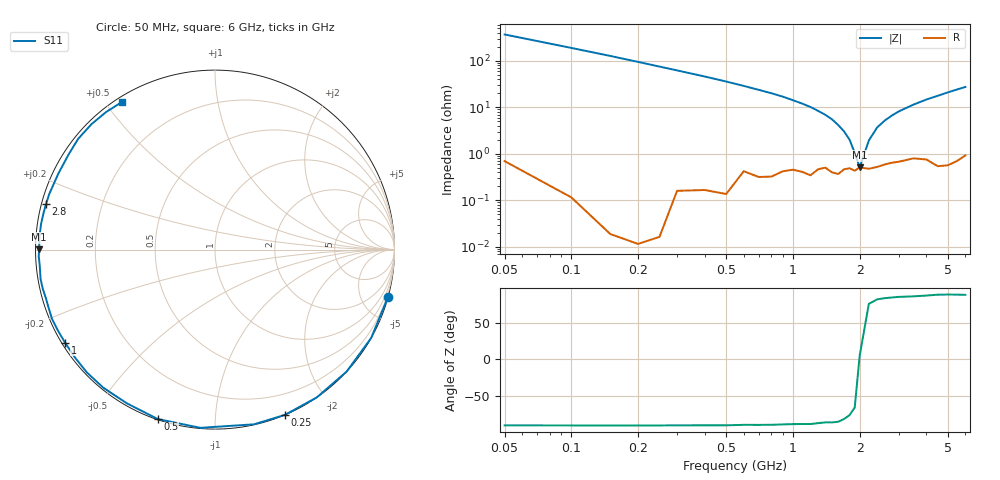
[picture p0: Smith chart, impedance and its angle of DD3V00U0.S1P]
! Infineon Technologies  Discrete & RF Semiconductors
! BBY58-02W
! Si Tuning Diode in SCD-80
! VR = 3 V
! S-Parameters:  June  2000
# GHz  S  MA  R  50
!  f  S11
! GHz  MAG  ANG
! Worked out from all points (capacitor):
!   34 points, 50 MHz to 6 GHz, reference 50 ohm
!   read as one part to ground: C = 8.36 pF near 50 MHz
!   lowest |Z| = 512 mohm at 2 GHz (marker M1)
!   series resonance near 1.996 GHz, so ESL is about 760 pH
!   S11 on the Smith chart (normalised r, x): 50 MHz: 0.01, -7.40; 250 MHz: 0.00, -1.51; 500 MHz: 0.00, -0.72; 1 GHz: 0.01, -0.28; 2.8 GHz: 0.01, +0.13; 6 GHz: 0.02, +0.55
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0.05  0.9995 -15.4
0.1  0.9997 -29.5
0.15  0.9999 -42.8
0.2  0.9999 -55.5
0.25  0.9998 -67.1
0.3  0.9975 -77.4
0.4  0.9964 -94.7
0.5  0.9964 -108.6
0.6  0.9874 -119.9
0.7  0.9897 -129.0
0.8  0.9889 -136.2
0.9  0.985 -142.5
1  0.9833 -148.2
1.1  0.9846 -152.9
1.2  0.9868 -157.0
1.3  0.982 -161.0
1.6  0.9855 -170.5
1.9  0.9828 -177.8
2  0.9798 179.9
2.4  0.9794 171.6
2.8  0.975 164.8
3  0.974 161.5
3.5  0.9701 154.2
4  0.9725 147.2
4.5  0.9809 141.0
5  0.9809 134.5
5.5  0.9775 128.3
6  0.972 122.4
